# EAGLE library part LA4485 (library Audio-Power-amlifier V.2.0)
The LA4485 is a 5 W, two-channel power amplifier IC that requires a minimum of external parts, making it ideal for radio cassette players and car stereo equipment. The LA4485 eliminates the need for bootstrap capacitors, negative feedback capacitors, and oscillation prevention CR parts, all of which were necessities for power ICs previously. All of these functions are now on chip, keeping the number of external parts to an absolute minimum. The LA4485 is part of the Power (Stylish Power) Series, and supports two modes: dual and BTL.
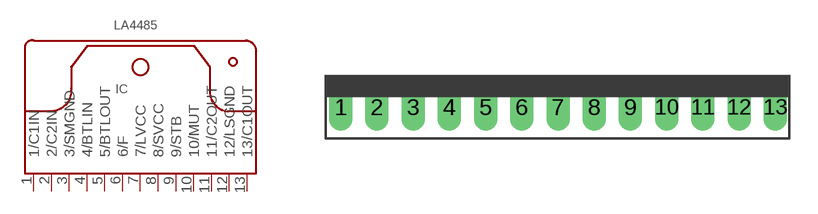
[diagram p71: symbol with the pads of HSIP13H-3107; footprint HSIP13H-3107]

Designator prefix IC

## LA4485  [HSIP13H-3107]
1  1/C1IN  in
2  2/C2IN  in
3  3/SMGND  pwr
4  4/BTLIN  in
5  5/BTLOUT  out
6  6/F
7  7/LVCC  pwr
8  8/SVCC  pwr
9  9/STB
10  10/MUT
11  11/C2OUT  out
12  12/LSGND  pwr
13  13/C1OUT  out

## Footprint HSIP13H-3107 (pad centres in mm)
drill 0.8 long: 1 -11.97,-1.27; 2 -9.97,-1.27; 3 -7.97,-1.27; 4 -5.97,-1.27; 5 -3.97,-1.27; 6 -1.97,-1.27; 7 0.03,-1.27; 8 2.03,-1.27; 9 4.03,-1.27; 10 6.03,-1.27; 11 8.03,-1.27; 12 10.03,-1.27; 13 12.03,-1.27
